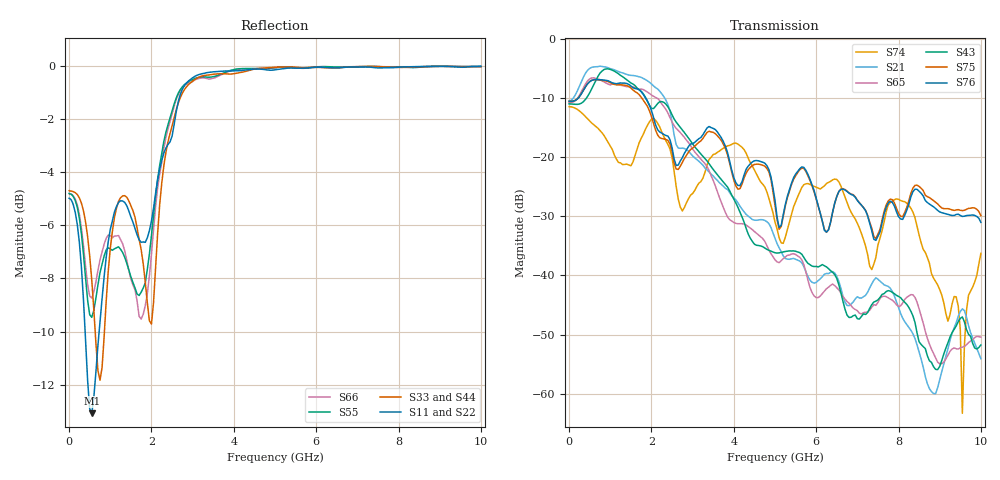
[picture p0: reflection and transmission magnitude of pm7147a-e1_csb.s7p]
# GHz S DB R 50
! S-Parameters data
! Freq  dbS11  angS11  dbS12  angS12  dbS13  angS13  dbS14  angS14
!  dbS15  angS15  dbS16  angS16  dbS17  angS17  dbS21  angS21
!  dbS22  angS22  dbS23  angS23  dbS24  angS24  dbS25  angS25
!  dbS26  angS26  dbS27  angS27  dbS31  angS31  dbS32  angS32
!  dbS33  angS33  dbS34  angS34  dbS35  angS35  dbS36  angS36
!  dbS37  angS37  dbS41  angS41  dbS42  angS42  dbS43  angS43
!  dbS44  angS44  dbS45  angS45  dbS46  angS46  dbS47  angS47
!  dbS51  angS51  dbS52  angS52  dbS53  angS53  dbS54  angS54
!  dbS55  angS55  dbS56  angS56  dbS57  angS57  dbS61  angS61
!  dbS62  angS62  dbS63  angS63  dbS64  angS64  dbS65  angS65
!  dbS66  angS66  dbS67  angS67  dbS71  angS71  dbS72  angS72
!  dbS73  angS73  dbS74  angS74  dbS75  angS75  dbS76  angS76
!  dbS77  angS77
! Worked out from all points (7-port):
!   279 points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, 1 Hz to 10 GHz, reference 50 ohm
!   strongest paths, dB at 1 Hz, 7.943 MHz, 3.05 GHz, 6.55 GHz, 10 GHz:
!     S76: -10.6, -10.6, -17.5, -25.8, -31.0
!     S75: -10.6, -10.6, -18.2, -25.8, -29.9
!     S43: -11.0, -11.0, -18.3, -41.6, -51.8
!     S65: -10.8, -10.8, -19.1, -42.4, -50.4
!     S21: -10.5, -10.5, -20.1, -41.0, -54.1
!     S74: -11.5, -11.5, -25.6, -24.2, -36.3
!   lowest |S11| = -13.1 dB at 550 MHz (marker M1), VSWR 1.57, Z = 31.9 - j0.816 ohm
!   |S11| at or under -10 dB: 388.8 MHz to 729.2 MHz (340.4 MHz wide, 60.9 % of centre)
